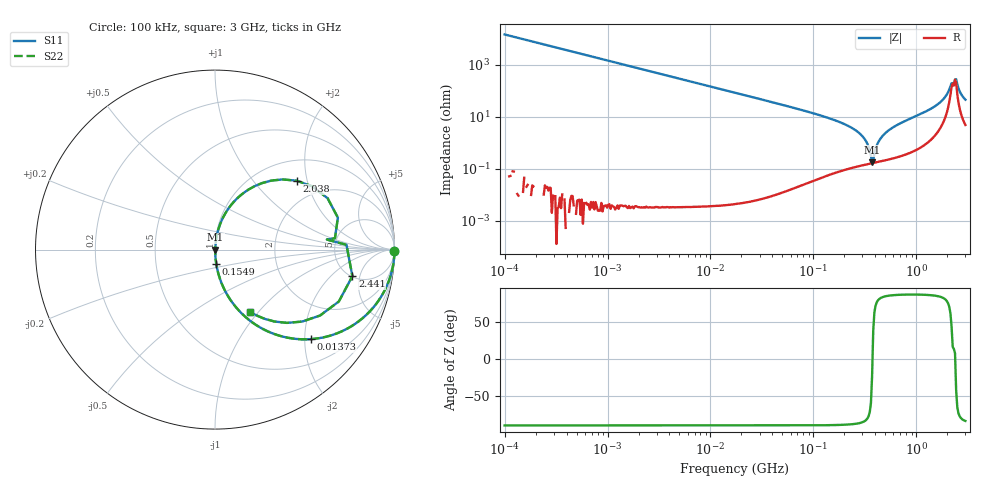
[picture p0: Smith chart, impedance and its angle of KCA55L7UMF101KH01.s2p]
!Murata Part Number: KCA55L7UMF101KH01
!These Parameters are Measured in Series Mode Connection
!Data Generated on Jan 08, 2026
!  o--ll--o
!Port1  Port2
!  o------o
!Operation Temp=25[degC], DC Bias Voltage=0[V]
!Freq. Start=100[kHz] Stop=3[GHz] 401[Steps]
# Hz S RI R 50
!Freq.(Hz) S11(Real) S11(Imag) S21(Real) S21(Imag) S12(Real) S12(Imag) S22(Real) S22(Imag)
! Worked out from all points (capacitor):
!   401 points, 100 kHz to 3 GHz, reference 50 ohm
!   read as one part in series: C = 108 pF near 105.3 kHz
!   lowest |Z| = 179 mohm at 372 MHz (marker M1)
!   series resonance near 375.4 MHz, so ESL is about 1.7 nH
!   S11 on the Smith chart (normalised r, x): 100 kHz: open; 13.73 MHz: 1.00, -2.14; 154.9 MHz: 1.00, -0.16; 2.038 GHz: 1.45, +1.73; 2.441 GHz: 5.10, -3.85; 3 GHz: 1.10, -0.91
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100000  1 -0.00679  4.61e-05 0.00679  4.61e-05 0.00679  1 -0.00679
562235  0.9985 -0.0381  0.00146 0.0381  0.00146 0.0381  0.9985 -0.0381
3161081  0.9559 -0.2052  0.0441 0.2052  0.0441 0.2052  0.9559 -0.2052
6674626  0.8295 -0.3761  0.1705 0.3761  0.1705 0.3761  0.8295 -0.3761
1.37349e7  0.5341 -0.4988  0.4659 0.4988  0.4659 0.4988  0.5341 -0.4988
1.77727e7  0.406 -0.491  0.594 0.491  0.594 0.491  0.406 -0.491
3.850681e7  0.1252 -0.3309  0.8748 0.3309  0.8748 0.3309  0.1252 -0.3309
9.738194e7  0.0198 -0.138  0.9802 0.138  0.9802 0.138  0.0198 -0.138
1.548634e8  0.0068 -0.0782  0.9932 0.0782  0.9932 0.0782  0.0068 -0.0782
2.874592e8  0.00176 -0.0212  0.9982 0.0212  0.9982 0.0212  0.00176 -0.0212
3.269943e8  0.00159 -0.0109  0.9984 0.0109  0.9984 0.0109  0.00159 -0.0109
3.719668e8  0.00164 -0.000712  0.9984 0.000712  0.9984 0.000712  0.00164 -0.000712
3.916425e8  0.00173 0.00338  0.9983 -0.00338  0.9983 -0.00338  0.00173 0.00338
4.455063e8  0.00211 0.0138  0.9979 -0.0138  0.9979 -0.0138  0.00211 0.0138
5.475153e8  0.0033 0.0314  0.9967 -0.0314  0.9967 -0.0314  0.0033 0.0314
1.495945e9  0.0713 0.2237  0.9287 -0.2237  0.9287 -0.2237  0.0713 0.2237
1.7917e9  0.1867 0.3345  0.8133 -0.3345  0.8133 -0.3345  0.1867 0.3345
2.038117e9  0.4548 0.3837  0.5452 -0.3837  0.5452 -0.3837  0.4548 0.3837
2.318426e9  0.6235 0.056  0.3765 -0.056  0.3765 -0.056  0.6235 0.056
2.441062e9  0.7655 -0.1479  0.2345 0.1479  0.2345 0.1479  0.7655 -0.1479
2.637286e9  0.4856 -0.4011  0.5144 0.4011  0.5144 0.4011  0.4856 -0.4011
3e9  0.1969 -0.3478  0.8031 0.3478  0.8031 0.3478  0.1969 -0.3478
